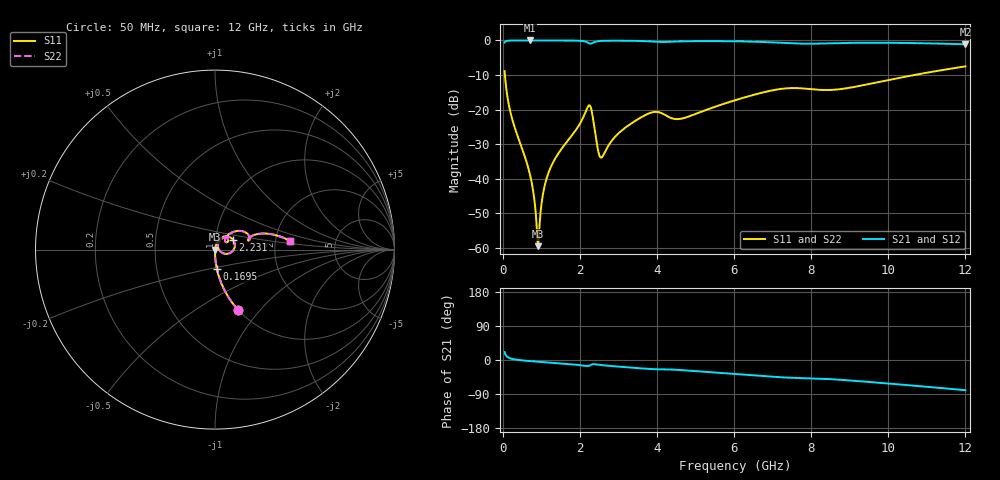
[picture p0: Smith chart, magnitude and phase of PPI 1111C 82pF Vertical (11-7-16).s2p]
# GHz S MA R 50
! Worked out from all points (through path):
!   1601 points, 50 MHz to 12 GHz, reference 50 ohm
!   highest |S21| = -0.01 dB at 707.2 MHz (marker M1); lowest = -1.1 dB at 12 GHz (marker M2)
!   group delay of S21, straight-line fit = 18.2 ps
!   lowest |S11| = -59.5 dB at 916.4 MHz (marker M3), VSWR 1.00, Z = 50.1 - j0.0159 ohm
!   |S11| at or under -10 dB: 57.72 MHz to 10.68 GHz (10.62 GHz wide, 198 % of centre)
!   |S22| runs from -59.5 to -7.5 dB; largest |S21 - S12| = 0
!   S11 on the Smith chart (normalised r, x): 50 MHz: 1.00, -0.77; 169.5 MHz: 1.00, -0.22; 2.231 GHz: 1.22, +0.13; 12 GHz: 2.42, +0.28
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0.05  0.3594 -69.1  0.9329 20.8  0.9329 20.8  0.3594 -69.1
0.1695  0.1095 -84.3  0.9935 5.4  0.9935 5.4  0.1095 -84.3
0.70725  0.01146 -88.3  0.999 -2.9  0.999 -2.9  0.01146 -88.3
0.7894062  0.006681 -85.2  0.999 -3.6  0.999 -3.6  0.006681 -85.2
0.8790313  0.002168 -66.0  0.9989 -4.3  0.9989 -4.3  0.002168 -66.0
0.916375  0.001053 -8.6  0.9989 -4.6  0.9989 -4.6  0.001053 -8.6
0.9537187  0.002015 52.8  0.9989 -4.9  0.9989 -4.9  0.002015 52.8
1.06575  0.006882 74.6  0.9987 -5.7  0.9987 -5.7  0.006882 74.6
1.215125  0.01328 77.5  0.9985 -6.8  0.9985 -6.8  0.01328 77.5
2.044156  0.06854 65.1  0.9847 -14.0  0.9847 -14.0  0.06854 65.1
2.230875  0.1144 28.5  0.9146 -15.7  0.9146 -15.7  0.1144 28.5
2.305563  0.09687 -6.0  0.9035 -12.0  0.9035 -12.0  0.09687 -6.0
2.469875  0.02637 -12.7  0.9735 -12.3  0.9735 -12.3  0.02637 -12.7
2.5595  0.02013 22.5  0.9835 -13.4  0.9835 -13.4  0.02013 22.5
3.149531  0.05297 62.9  0.9906 -18.6  0.9906 -18.6  0.05297 62.9
4.038312  0.09167 37.2  0.9531 -24.5  0.9531 -24.5  0.09167 37.2
4.605937  0.07329 40.1  0.9683 -26.5  0.9683 -26.5  0.07329 40.1
6.025  0.1361 45.0  0.9715 -37.0  0.9715 -37.0  0.1361 45.0
7.182656  0.1974 28.2  0.926 -45.5  0.926 -45.5  0.1974 28.2
8.019156  0.1966 15.1  0.8962 -48.4  0.8962 -48.4  0.1966 15.1
10.01331  0.2679 19.4  0.9241 -62.2  0.9241 -62.2  0.2679 19.4
12  0.4215 6.5  0.8784 -79.7  0.8784 -79.7  0.4215 6.5
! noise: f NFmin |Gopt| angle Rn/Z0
0.05  0.0003855  0.8705  0.4627  0.0006409
1.372  0.004452  0.718  6.777  0.003112
2.701  0.01614  0.8375  13.38  0.02073
4.031  0.04061  0.9016  19.83  0.08772
5.36  0.02868  0.8255  26.06  0.0328
6.682  0.04447  0.8602  32.16  0.06295
8.012  0.08158  0.9087  38.18  0.1755
9.341  0.0647  0.8723  43.84  0.09405
10.67  0.05616  0.8402  49.18  0.06165
12  0.05472  0.8237  54.25  0.05174
